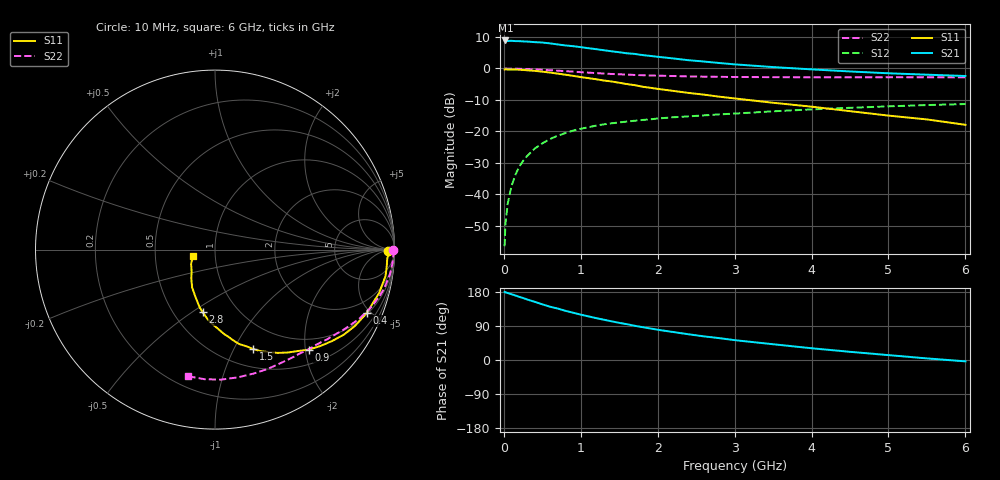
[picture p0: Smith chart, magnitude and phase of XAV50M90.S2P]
! SIEMENS Discrete & RF Semiconductors
! BFY180
! Si NPN RF Bipolar Junction Transistor in MICRO-X
! VCE = 0.5 V  IC = 0.9 mA
! Common Emitter S-Parameters:  May  1997
# GHz  S  MA  R  50
!  f  S11  S21  S12  S22
! GHz  MAG  ANG  MAG  ANG  MAG  ANG  MAG  ANG
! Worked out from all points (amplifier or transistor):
!   36 points, 10 MHz to 6 GHz, reference 50 ohm
!   highest |S21| = 8.9 dB at 20 MHz (marker M1)
!   |S21| within 3 dB of that: start of sweep to 1.267 GHz
!   unconditionally stable (mu >= 1): 2.279 GHz to end of sweep
!   at 250 MHz: K = 0.12, MSG = 19.0 dB, |S12| = -29.4 dB
!   at 1.4 GHz: K = 0.72, MSG = 11.4 dB, |S12| = -17.4 dB
!   at 6 GHz: K = 1.26, MAG = 1.4 dB, |S12| = -11.3 dB
!   S11 on the Smith chart (normalised r, x): 10 MHz: 52, -10; 400 MHz: 1.09, -4.77; 900 MHz: 0.77, -2.07; 1.5 GHz: 0.70, -1.19; 2.8 GHz: 0.69, -0.55; 6 GHz: 0.78, -0.05
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0.01  0.9634 -0.4  2.74 179.7  0.0015 85.7  0.9925 -0.2
0.02  0.969 -1.4  2.785 178.6  0.0033 93.8  0.995 -0.6
0.05  0.9612 -2.9  2.729 176.9  0.0071 86.7  0.9934 -1.7
0.1  0.9615 -5.9  2.752 173.5  0.0136 86.8  0.993 -3.3
0.15  0.9613 -8.9  2.721 170.2  0.0204 83.7  0.9904 -4.9
0.25  0.9466 -14.7  2.691 163.6  0.0339 80.2  0.9841 -8.2
0.3  0.9352 -17.1  2.676 159.9  0.0403 77.0  0.9773 -9.7
0.4  0.9163 -22.6  2.619 153.6  0.053 73.8  0.968 -12.7
0.5  0.8893 -28.4  2.583 146.9  0.0645 69.5  0.9537 -15.7
0.6  0.8604 -33.4  2.502 140.6  0.0756 66.2  0.9375 -18.4
0.9  0.7633 -46.9  2.258 124.8  0.1031 56.6  0.8905 -25.7
1.1  0.7013 -54.9  2.096 115.1  0.1166 51.5  0.858 -29.9
1.5  0.5928 -69.0  1.811 98.0  0.1387 43.3  0.8076 -37.2
1.8  0.5131 -78.9  1.633 86.8  0.1518 39.3  0.7811 -41.9
2  0.4735 -83.8  1.533 79.8  0.1602 36.7  0.7686 -44.9
2.2  0.4403 -88.0  1.443 73.9  0.1675 34.0  0.7581 -48.0
2.6  0.3839 -96.9  1.289 62.4  0.1796 30.2  0.7416 -53.5
2.8  0.3561 -101.0  1.22 57.7  0.1862 28.5  0.7362 -56.2
3.5  0.2849 -112.5  1.051 41.6  0.2084 22.7  0.727 -65.9
4.5  0.2096 -129.1  0.896 21.6  0.237 13.8  0.723 -79.9
5.5  0.155 -149.2  0.796 4.2  0.2618 4.6  0.7246 -94.6
6  0.1272 -164.4  0.759 -3.6  0.272 -0.1  0.7211 -101.9
